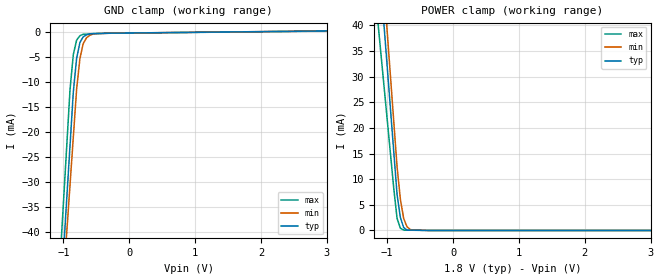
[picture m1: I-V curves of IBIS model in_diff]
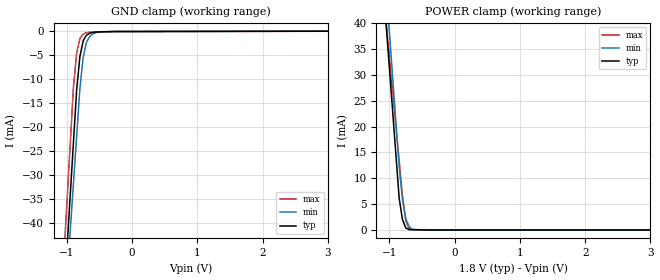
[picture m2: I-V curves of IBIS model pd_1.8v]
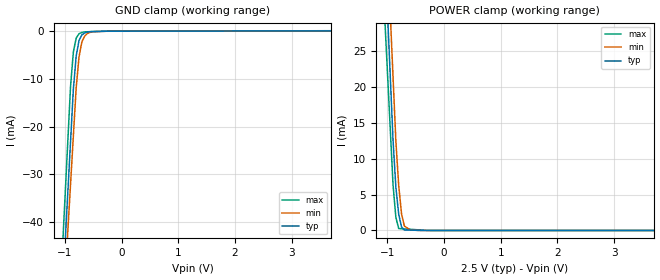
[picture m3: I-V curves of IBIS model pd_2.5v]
|Texas Instruments Incorporated
|AFE0707
[IBIS Ver] 4.0
[File Name] afe7070.ibs
[File Rev] 3.0
[Date]   03-14-2011
[Notes]  Quality Check of this IBIS model: Model Passes IBIS Check. Model
   parses into ICX IS. Simulates with Hyperlynx.
   1. MIN TYP MAX information is based on Temperature and Voltage
   characteristics only.
   2. Package information extracted using Tektronix IConnect Software.
[Disclaimer]
  This model is designed as an aid for customers of Texas Instruments.
  TI and its licensors and suppliers make no warranties, either expressed
  or implied, with respect to this model, including the warranties of
  merchantability or fitness for a particular purpose.  The model is
  provided solely on an "as is" basis.  The entire risk as to its quality
  and performance is with the customer.
[Copyright] (C) Copyright 2012 Texas Instruments Incorporated.
   All rights reserved.
[Component] AFE7070
[Manufacturer] TI
[Package]
| variable   typ   min   max
R_pkg  1.000E-02   1.000E-02   1.000E-02
L_pkg  2.875E-09   2.600E-09   3.150E-09
C_pkg  6.167E-13   5.550E-13   6.783E-13
[Pin] signal_name  model_name  R_pin  L_pin C_pin
1   DACCLKP   in_diff   1.000E-02   3.150E-09   6.783E-13
2   DACCLKN   in_diff   1.000E-02   3.040E-09   6.537E-13
3   CLKVDD   POWER   1.000E-02   2.930E-09   6.290E-13
4   DACVDD   POWER   1.000E-02   2.820E-09   6.043E-13
5   CLKIO   out_io   1.000E-02   2.710E-09   5.797E-13
6   IQFLAG   in_pd   1.000E-02   2.600E-09   5.550E-13
7   SYNC_SLEEP  in_pd   1.000E-02   2.600E-09   5.550E-13
8   RESETB   in_pu   1.000E-02   2.710E-09   5.797E-13
9   D13   in_pd   1.000E-02   2.820E-09   6.043E-13
10  D12   in_pd   1.000E-02   2.930E-09   6.290E-13
11  GND   GND   1.000E-02   3.040E-09   6.537E-13
12  DVDD   POWER   1.000E-02   3.150E-09   6.783E-13
13  IOVDD   POWER   1.000E-02   3.150E-09   6.783E-13
14  D11   in_pd   1.000E-02   3.040E-09   6.537E-13
15  D10   in_pd   1.000E-02   2.930E-09   6.290E-13
16  D9   in_pd   1.000E-02   2.820E-09   6.043E-13
17  D8   in_pd   1.000E-02   2.710E-09   5.797E-13
18  D7   in_pd   1.000E-02   2.600E-09   5.550E-13
19  D6   in_pd   1.000E-02   2.600E-09   5.550E-13
20  D5   in_pd   1.000E-02   2.710E-09   5.797E-13
21  D4   in_pd   1.000E-02   2.820E-09   6.043E-13
22  D3   in_pd   1.000E-02   2.930E-09   6.290E-13
23  D2   in_pd   1.000E-02   3.040E-09   6.537E-13
24  IOVDD   POWER   1.000E-02   3.150E-09   6.783E-13
25  DVDD   POWER   1.000E-02   3.150E-09   6.783E-13
26  GND   GND   1.000E-02   3.040E-09   6.537E-13
27  D1   in_pd   1.000E-02   2.930E-09   6.290E-13
28  D0   in_pd   1.000E-02   2.820E-09   6.043E-13
29  SDIO   out_io   1.000E-02   2.710E-09   5.797E-13
30  SCLK   in_pd   1.000E-02   2.600E-09   5.550E-13
31  SDENB   in_pu   1.000E-02   2.600E-09   5.550E-13
32  LO_P   term   1.000E-02   2.710E-09   5.797E-13
33  LO_N   term   1.000E-02   2.820E-09   6.043E-13
34  ALARM_SDO   out_tri   1.000E-02   2.930E-09   6.290E-13
35  TESTMODE   GND   1.000E-02   3.040E-09   6.537E-13
36  ATEST   NC   1.000E-02   3.150E-09   6.783E-13
37  DACVDDB   POWER   1.000E-02   3.150E-09   6.783E-13
38  MODVDD   POWER   1.000E-02   3.040E-09   6.537E-13
39  MODVDD   POWER   1.000E-02   2.930E-09   6.290E-13
40  FUSEVDD   POWER   1.000E-02   2.820E-09   6.043E-13
41  GND   GND   1.000E-02   2.710E-09   5.797E-13
42  RFOUT   term   1.000E-02   2.600E-09   5.550E-13
43  GND   GND   1.000E-02   2.600E-09   5.550E-13
44  LVDSN   out_lvds  1.000E-02   2.710E-09   5.797E-13
45  LVDSP   out_lvds  1.000E-02   2.820E-09   6.043E-13
46  LVDSVDD   POWER   1.000E-02   2.930E-09   6.290E-13
47  BG_BYP   term   1.000E-02   3.040E-09   6.537E-13
48  DACVDDA   POWER   1.000E-02   3.150E-09   6.783E-13
[Diff Pin] inv_pin vdiff tdelay_typ tdelay_min tdelay_max
1   2   350mV NA   NA   NA
45   44   NA   NA   NA   NA
[Model selector] in_pd
pd_1.8v   cmos input w/int pull down,iovdd=1.8v
pd_2.5v   cmos input w/int pull down,iovdd=2.5v
pd_3.3v   cmos input w/int pull down,iovdd=3.3v
[Model selector] in_pu
pu_1.8v   cmos input w/int pull up,iovdd=1.8v
pu_2.5v   cmos input w/int pull up,iovdd=2.5v
pu_3.3v   cmos input w/int pull up,iovdd=3.3v
[Model selector] out_io
io_1.8v   cmos bidir w/int pull down,iovdd=1.8v
io_2.5v   cmos bidir w/int pull down,iovdd=2.5v
io_3.3v   cmos bidir w/int pull down,iovdd=3.3v
[Model selector] out_tri
tri_1.8v  cmos 3-state output,iovdd=1.8v
tri_2.5v  cmos 3-state output,iovdd=2.5v
tri_3.3v  cmos 3-state output,iovdd=3.3v
[Model]  term
Model_type Terminator
C_comp   0   0   0
[Voltage Range]  3.30  3.00  3.60
[Temperature Range] 25   85   -40
| Models and submodels in the file (15): in_diff (Input), pd_1.8v (Input), pd_2.5v (Input), pd_3.3v (Input), pu_1.8v (Input), pu_2.5v (Input), pu_3.3v (Input), io_1.8v (I/O), tri_1.8v (3-state), io_2.5v (I/O), tri_2.5v (3-state), io_3.3v (I/O), tri_3.3v (3-state), out_lvds (3-state), term (Terminator)
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[Model] in_diff
Model_type Input
Vinl = 1.07500V
Vinh = 1.42500V
C_comp 479.000fF 475.000fF 483.000fF
| variable typ   min   max
[Voltage Range] 1.80000V 1.71000V 1.89000V
[POWER Clamp Reference] 1.80000V 1.71000V 1.89000V
[GND Clamp Reference] 0.00000V 0.00000V 0.00000V
[Temperature Range] 25   85   -40
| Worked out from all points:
|   GND clamp passes 1 mA (typ) near -0.70 V on its own axis
|   POWER clamp passes 1 mA (typ) near -0.76 V on its own axis
[GND Clamp]
-1.8V     -215.2mA   -202.5mA   -215mA
-900mV    -22.64mA   -30.51mA   -11.45mA
-850mV    -11.94mA   -20.95mA   -4.488mA
-800mV    -5.261mA   -11.4mA    -1.606mA
-750mV    -2.088mA   -5.294mA   -720.1uA
-700mV    -943.5uA   -2.307mA   -437.6uA
-650mV    -551.6uA   -1.156mA   -409.3uA
-600mV    -368.4uA   -623uA     -380.9uA
-500mV    -276.8uA   -298.8uA   -324.2uA
3.6V      314.4uA    309.6uA    283.2uA
[POWER Clamp]
-1.8V     165.2mA    179.5mA    129.4mA
-950mV    23.66mA    30mA       14.91mA
-900mV    15.34mA    21.21mA    8.176mA
-850mV    7.017mA    12.41mA    2.338mA
-800mV    2.537mA    6.12mA     446.7uA
-750mV    569.4uA    2.357mA    69.52uA
-700mV    84.92uA    733.1uA    61.14uA
-650mV    72.79uA    176.7uA    52.77uA
-600mV    60.66uA    83.78uA    44.39uA
3.6V      0A         0A         0A
[Model] pd_1.8v
Model_type Input
Vinl = 540.000mV
Vinh = 1.25000V
C_comp 542.000fF 490.000fF 594.000fF
| variable typ   min   max
[Voltage Range] 1.80000V 1.71000V 1.89000V
[POWER Clamp Reference] 1.80000V 1.71000V 1.89000V
[GND Clamp Reference] 0.00000V 0.00000V 0.00000V
[Temperature Range] 25   85   -40
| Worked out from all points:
|   GND clamp passes 1 mA (typ) near -0.71 V on its own axis
|   POWER clamp passes 1 mA (typ) near -0.77 V on its own axis
[GND Clamp]
-1.8V     -224.9mA   -212.5mA   -229.1mA
-900mV    -23.31mA   -31.86mA   -11.74mA
-850mV    -12.11mA   -21.83mA   -4.442mA
-800mV    -5.17mA    -11.79mA   -1.457mA
-750mV    -1.934mA   -5.364mA   -544.7uA
-700mV    -773.9uA   -2.237mA   -255.1uA
-650mV    -375.2uA   -1.031mA   -147.5uA
-600mV    -184.9uA   -469.2uA   -126.6uA
-500mV    -79.55uA   -112.6uA   -84.79uA
3.6V      75.87uA    88.88uA    62.25uA
[POWER Clamp]
-1.8V     166mA      177.6mA    140.5mA
-950mV    22.97mA    29.6mA     26.75mA
-850mV    6.144mA    12.18mA    13.37mA
-800mV    2.036mA    5.963mA    6.681mA
-750mV    421.1uA    2.274mA    1.801mA
-700mV    59.77uA    692.6uA    324.9uA
-650mV    51.23uA    154.1uA    57.8uA
-350mV    0A         0A         14.99uA
3.6V      0A         0A         0A
[Model] pd_2.5v
Model_type Input
Vinl = 750.000mV
Vinh = 1.75000V
C_comp 542.000fF 490.000fF 594.000fF
| variable typ   min   max
[Voltage Range] 2.50000V 2.25000V 2.75000V
[POWER Clamp Reference] 2.50000V 2.25000V 2.75000V
[GND Clamp Reference] 0.00000V 0.00000V 0.00000V
[Temperature Range] 25   85   -40
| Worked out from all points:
|   GND clamp passes 1 mA (typ) near -0.71 V on its own axis
|   POWER clamp passes 1 mA (typ) near -0.76 V on its own axis
[GND Clamp]
-2.5V     -377.5mA   -357.5mA   -393.8mA
-900mV    -23.2mA    -32.14mA   -11.61mA
-850mV    -12.13mA   -21.97mA   -4.372mA
-800mV    -5.183mA   -11.8mA    -1.432mA
-750mV    -1.938mA   -5.374mA   -536.1uA
-700mV    -775.5uA   -2.243mA   -252uA
-650mV    -375.9uA   -1.034mA   -146.2uA
-600mV    -185.1uA   -470.9uA   -125.3uA
-500mV    -79.43uA   -112.9uA   -83.71uA
-250mV    -9.015uA   -9.698uA   -8.861uA
5V        101.9uA    95.08uA    131.3uA
[POWER Clamp]
-2.5V     304.1mA    309.1mA    261.7mA
-1.05V    39.96mA    48.44mA    30.31mA
-900mV    12.63mA    21.47mA    6.371mA
-850mV    6.042mA    12.48mA    1.825mA
-800mV    2.262mA    6.296mA    268.5uA
-750mV    492.8uA    2.328mA    243uA
-700mV    71.82uA    618.8uA    217.4uA
-600mV    51.3uA     93.79uA    166.2uA
-200mV    0A         0A         0A
5V        0A         0A         0A
